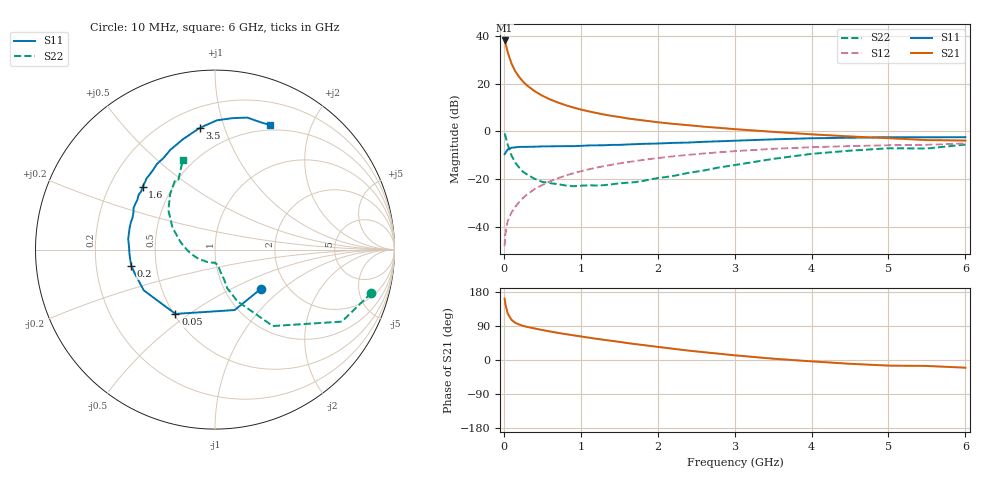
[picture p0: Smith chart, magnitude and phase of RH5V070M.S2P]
! SIEMENS Small Signal Semiconductors
! BFR106
! Si NPN RF Bipolar Junction Transistor in SOT23
! VCE = 5 V  IC = 70 mA
! Common Emitter S-Parameters:  August  1996
# GHz  S  MA  R  50
!  f  S11  S21  S12  S22
! GHz  MAG  ANG  MAG  ANG  MAG  ANG  MAG  ANG
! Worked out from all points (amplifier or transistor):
!   36 points, 10 MHz to 6 GHz, reference 50 ohm
!   highest |S21| = 38.0 dB at 10 MHz (marker M1)
!   |S21| within 3 dB of that: start of sweep to 35.18 MHz
!   unconditionally stable (mu >= 1): 216.1 MHz to 2.354 GHz
!   at 250 MHz: K = 1.03, MAG = 23.3 dB, |S12| = -27.8 dB
!   at 1.4 GHz: K = 1.06, MAG = 8.8 dB, |S12| = -13.9 dB
!   at 6 GHz: K = 0.99, MSG = 0.6 dB, |S12| = -5.0 dB
!   S11 on the Smith chart (normalised r, x): 10 MHz: 1.47, -0.73; 50 MHz: 0.51, -0.44; 200 MHz: 0.36, -0.08; 1.6 GHz: 0.34, +0.33; 3.5 GHz: 0.33, +0.83; 6 GHz: 0.44, +1.44
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0.01  0.3365 -40.5  79.8 161.9  0.004 81.3  0.904 -15.5
0.02  0.3541 -72.0  70.65 147.8  0.0071 67.1  0.8124 -29.6
0.05  0.4206 -121.6  45.42 122.4  0.0135 62.2  0.5339 -52.9
0.1  0.4572 -150.2  26.18 105.9  0.0203 62.8  0.3123 -66.7
0.15  0.4652 -162.6  17.95 98.0  0.0267 67.1  0.2231 -72.5
0.2  0.4752 -168.9  13.69 93.6  0.0336 69.6  0.1749 -73.0
0.25  0.4757 -173.5  10.98 90.0  0.0408 71.1  0.143 -74.9
0.3  0.477 -176.8  9.197 87.5  0.0479 72.5  0.1268 -76.4
0.4  0.48 177.4  6.968 83.2  0.0624 73.1  0.1022 -77.8
0.5  0.4869 173.2  5.588 79.1  0.0762 73.2  0.0884 -78.8
0.6  0.4883 169.3  4.682 75.3  0.0908 72.3  0.0833 -81.5
0.8  0.4926 162.1  3.552 68.4  0.1194 70.3  0.0744 -89.4
0.9  0.4923 159.1  3.172 65.3  0.1335 69.1  0.0717 -91.8
1.1  0.51 152.8  2.639 59.1  0.161 66.6  0.0749 -102.4
1.3  0.5143 147.2  2.261 53.3  0.1883 63.6  0.0752 -112.3
1.6  0.5336 139.0  1.881 44.9  0.2273 59.3  0.0847 -129.2
2.2  0.5765 124.0  1.441 29.7  0.3017 50.3  0.1172 -160.1
2.8  0.6224 110.2  1.189 16.5  0.3673 41.1  0.1769 173.3
3.5  0.6835 97.1  0.982 3.5  0.4335 30.6  0.2669 152.6
4.5  0.7383 82.6  0.786 -10.0  0.4937 16.0  0.3963 129.2
5.5  0.7536 70.0  0.66 -15.7  0.5263 6.4  0.4402 117.6
6  0.7589 66.2  0.645 -20.3  0.562 -0.6  0.532 109.6
